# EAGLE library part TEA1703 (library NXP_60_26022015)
GreenChip SMPS standby control IC The TEA1703T is a low power standby controller IC intended to be used in applications which require an extreme low no-load standby power. The TEA1703T includes circuitry for detecting output voltage, output power and switching. The TEA1703T integrates a switched-mode optocoupler driver, which enables an optocoupler to be driven with a high peak current while keeping the required power low1 . The TEA1703T’s typical current consumption is 30 μA. In a typical notebook adapter application the TEA1703T’s power consumption is less than 0.5 mW. AAL Eindhoven MK
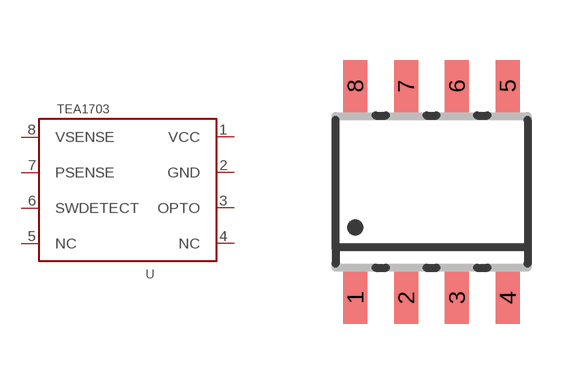
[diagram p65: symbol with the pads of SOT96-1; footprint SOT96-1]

Designator prefix U

## TEA1703  [SOT96-1]
1  VCC  pwr
2  GND  pwr
3  OPTO  out
4  NC  in
5  NC  in
6  SWDETECT  pas
7  PSENSE  pas
8  VSENSE  pas

## Footprint SOT96-1 (pad centres in mm)
SOT96-1 SO8: plastic small outline package; 8 leads; body width 3.9 mm JEDEC: MS-012 IEC: 076E03
smd 0.6 x 1.3: 1 -1.905,-2.65; 2 -0.635,-2.65; 3 0.635,-2.65; 4 1.905,-2.65; 5 1.905,2.65; 6 0.635,2.65; 7 -0.635,2.65; 8 -1.905,2.65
